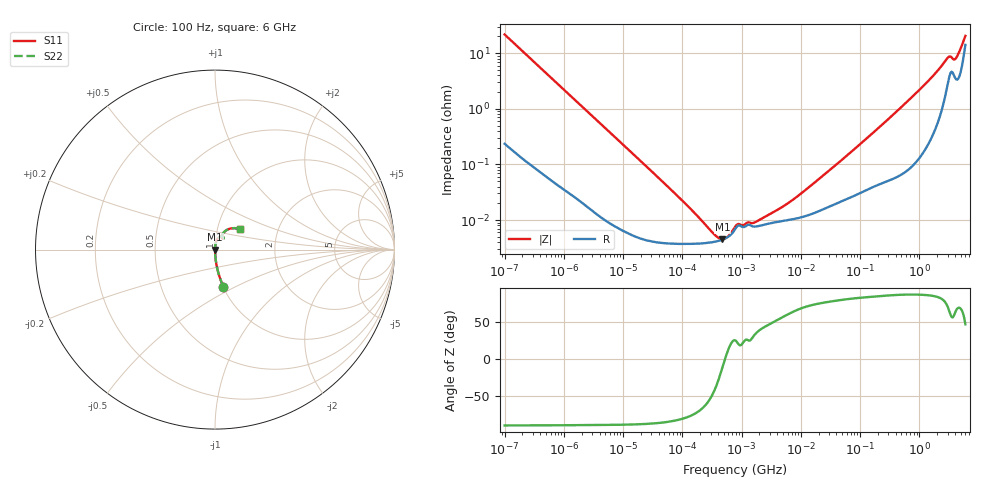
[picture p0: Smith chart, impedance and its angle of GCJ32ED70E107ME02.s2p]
!Murata Part Number: GCJ32ED70E107ME02
!These Parameters are Measured in Series Mode Connection
!Data Generated on Mar 13, 2026
!  o--ll--o
!Port1  Port2
!  o------o
!Operation Temp=25[degC], DC Bias Voltage=0[V]
!Freq. Start=100[Hz] Stop=6[GHz] 401[Steps]
# Hz S RI R 50
!Freq.(Hz) S11(Real) S11(Imag) S21(Real) S21(Imag) S12(Real) S12(Imag) S22(Real) S22(Imag)
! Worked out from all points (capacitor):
!   401 points, 100 Hz to 6 GHz, reference 50 ohm
!   read as one part in series: C = 73.1 uF near 109 Hz
!   lowest |Z| = 4.52 mohm at 473.3 kHz (marker M1)
!   series resonance near 525.6 kHz, so ESL is about 1.3 nH
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100  0.0471 -0.2065  0.9529 0.2065  0.9529 0.2065  0.0471 -0.2065
187  0.0147 -0.1147  0.9853 0.1147  0.9853 0.1147  0.0147 -0.1147
350  0.00469 -0.0622  0.9953 0.0622  0.9953 0.0622  0.00469 -0.0622
2008  0.000329 -0.0111  0.9997 0.0111  0.9997 0.0111  0.000329 -0.0111
40335  3.95e-05 -0.000562  1 0.000562  1 0.000562  3.95e-05 -0.000562
202169  3.79e-05 -9.62e-05  1 9.62e-05  1 9.62e-05  3.79e-05 -9.62e-05
231233  3.83e-05 -7.97e-05  1 7.97e-05  1 7.97e-05  3.83e-05 -7.97e-05
473344  4.43e-05 -9.2e-06  1 9.2e-06  1 9.2e-06  4.43e-05 -9.2e-06
774597  6.79e-05 3.21e-05  0.9999 -3.21e-05  0.9999 -3.21e-05  6.79e-05 3.21e-05
1813585  7.68e-05 5.56e-05  0.9999 -5.56e-05  0.9999 -5.56e-05  7.68e-05 5.56e-05
2169299  8.01e-05 6.89e-05  0.9999 -6.89e-05  0.9999 -6.89e-05  8.01e-05 6.89e-05
5809218  9.88e-05 0.000167  0.9999 -0.000167  0.9999 -0.000167  9.88e-05 0.000167
1.555665e7  0.000129 0.000414  0.9999 -0.000414  0.9999 -0.000414  0.000129 0.000414
6.233367e7  0.000244 0.00147  0.9998 -0.00147  0.9998 -0.00147  0.000244 0.00147
3.124326e8  0.000561 0.00677  0.9994 -0.00677  0.9994 -0.00677  0.000561 0.00677
1.309207e9  0.00282 0.0288  0.9972 -0.0288  0.9972 -0.0288  0.00282 0.0288
2.931063e9  0.0287 0.0721  0.9713 -0.0721  0.9713 -0.0721  0.0287 0.0721
3.205649e9  0.0415 0.0727  0.9585 -0.0727  0.9585 -0.0727  0.0415 0.0727
3.8344e9  0.0426 0.0602  0.9574 -0.0602  0.9574 -0.0602  0.0426 0.0602
4.193612e9  0.0378 0.0697  0.9622 -0.0697  0.9622 -0.0697  0.0378 0.0697
5.016141e9  0.0559 0.1027  0.9441 -0.1027  0.9441 -0.1027  0.0559 0.1027
6e9  0.1381 0.1125  0.8619 -0.1125  0.8619 -0.1125  0.1381 0.1125
